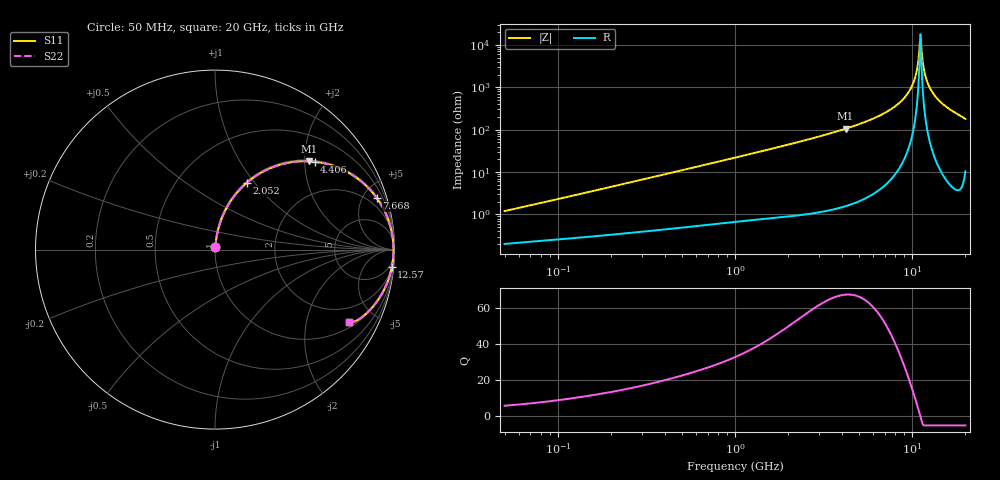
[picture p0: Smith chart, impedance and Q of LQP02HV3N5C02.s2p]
!Murata Part Number: LQP02HV3N5C02
!These Parameters are Measured in Series Mode Connection
!  o--[Z]--o
!Port1  Port2
!  o-------o
!Freq. Start=50[MHz] Stop=20[GHz], 401[Steps]
# Hz S RI R 50
!Freq.(Hz) S11(Real) S11(Imag) S21(Real) S21(Imag) S12(Real) S12(Imag) S22(Real) S22(Imag)
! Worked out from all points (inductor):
!   401 points, 50 MHz to 20 GHz, reference 50 ohm
!   read as one part in series: L = 3.72 nH near 51.52 MHz
!   highest Q = 67.2 at 4.212 GHz (marker M1), where L = 3.98 nH
!   self-resonance near 10.99 GHz
!   S11 on the Smith chart (normalised r, x): 50 MHz: 1.00, +0.02; 2.052 GHz: 1.02, +0.91; 4.406 GHz: 1.03, +2.24; 7.668 GHz: 1.14, +6.22; 12.57 GHz: 2, -20; 20 GHz: 1.21, -3.55
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5e7  0.00215 0.0118  0.9978 -0.0118  0.9978 -0.0118  0.00215 0.0118
1.364002e8  0.00381 0.0307  0.9962 -0.0307  0.9962 -0.0307  0.00381 0.0307
3.721004e8  0.0109 0.0809  0.9891 -0.0809  0.9891 -0.0809  0.0109 0.0809
1e9  0.0513 0.2059  0.9487 -0.2059  0.9487 -0.2059  0.0513 0.2059
2.05233e9  0.1775 0.3723  0.8225 -0.3723  0.8225 -0.3723  0.1775 0.3723
2.728004e9  0.2829 0.442  0.7171 -0.442  0.7171 -0.442  0.2829 0.442
4.212059e9  0.5254 0.492  0.4746 -0.492  0.4746 -0.492  0.5254 0.492
4.405649e9  0.5551 0.4896  0.4449 -0.4896  0.4449 -0.4896  0.5551 0.4896
7.442007e9  0.8867 0.3065  0.1133 -0.3065  0.1133 -0.3065  0.8867 0.3065
7.668323e9  0.9012 0.2874  0.0988 -0.2874  0.0988 -0.2874  0.9012 0.2874
8.907419e9  0.9594 0.1811  0.0406 -0.1811  0.0406 -0.1811  0.9594 0.1811
9.892087e9  0.9841 0.0985  0.0159 -0.0985  0.0159 -0.0985  0.9841 0.0985
1.034674e10  0.9903 0.0619  0.00973 -0.0619  0.00973 -0.0619  0.9903 0.0619
1.066139e10  0.9928 0.0372  0.00716 -0.0372  0.00716 -0.0372  0.9928 0.0372
1.082228e10  0.9937 0.0248  0.00635 -0.0248  0.00635 -0.0248  0.9937 0.0248
1.115139e10  0.9943 -0.000101  0.00565 0.000101  0.00565 0.000101  0.9943 -0.000101
1.149051e10  0.9938 -0.025  0.00621 0.025  0.00621 0.025  0.9938 -0.025
1.166392e10  0.993 -0.0374  0.00696 0.0374  0.00696 0.0374  0.993 -0.0374
1.201863e10  0.9906 -0.0622  0.00939 0.0622  0.00939 0.0622  0.9906 -0.0622
1.257102e10  0.9846 -0.0991  0.0154 0.0991  0.0154 0.0991  0.9846 -0.0991
1.504638e10  0.9337 -0.2387  0.0663 0.2387  0.0663 0.2387  0.9337 -0.2387
2e10  0.7477 -0.406  0.2523 0.406  0.2523 0.406  0.7477 -0.406
